PROGRAM EAP
VAR
	iEncode_Master AT %I*	:UDINT;
	iCount AT %I*	:UDINT;
	bWatchdog AT %I*	:BOOL;
	bEnable AT %I*	:BOOL;
	bReset AT %I*	:BOOL;
	fbTON_WD1: TON;
	fbTON_WD2: TON;
	// 通信超时错误
	bComTimeoutError: BOOL;
	
END_VAR

fbTON_WD1(IN:=bWatchdog , PT:=T#500MS , Q=> , ET=> );
fbTON_WD2(IN:=NOT bWatchdog , PT:=T#500MS , Q=> , ET=> );
IF fbTON_WD1.Q OR fbTON_WD2.Q THEN
	bComTimeoutError:=TRUE;
END_IF
IF bReset THEN
	bComTimeoutError:=FALSE;
END_IF

END_PROGRAM
